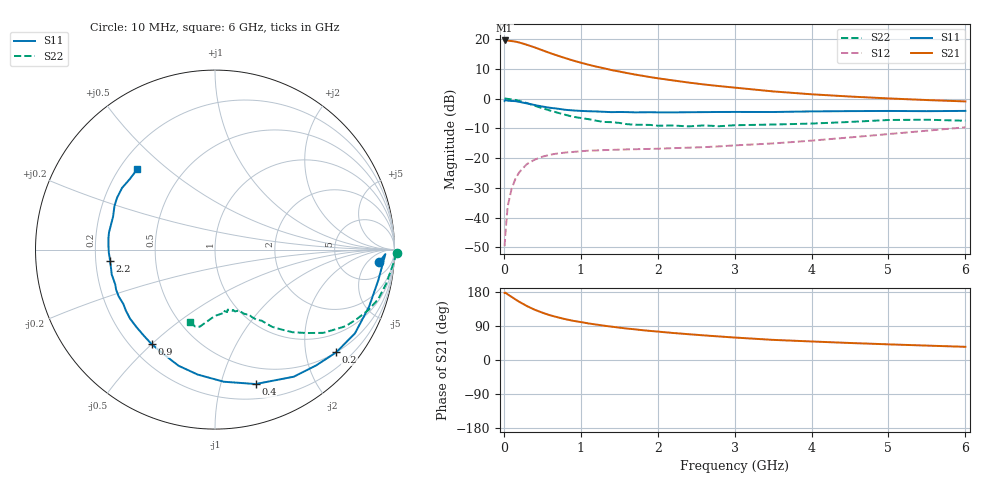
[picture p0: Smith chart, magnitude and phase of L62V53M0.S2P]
!  INFINEON TECHNOLOGIES Small Signal Semiconductors
! BFR380L3 , Si-NPN RF-Transistor in TSLP-3-1
!  Vce=2.5 V,  Ic=3 mA
! Common Emitter S-Parameters:  07. March 2005
#  GHz  S  MA  R  50
! f  S11  S21  S12  S22
! GHz  Mag  Ang  Mag  Ang  Mag  Ang  Mag  Ang
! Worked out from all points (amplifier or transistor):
!   36 points, 10 MHz to 6 GHz, reference 50 ohm
!   highest |S21| = 19.6 dB at 10 MHz (marker M1)
!   |S21| within 3 dB of that: start of sweep to 470 MHz
!   unconditionally stable (mu >= 1): 2.64 GHz to 4.677 GHz
!   at 250 MHz: K = 0.12, MSG = 20.9 dB, |S12| = -23.3 dB
!   at 1.4 GHz: K = 0.64, MSG = 13.4 dB, |S12| = -17.2 dB
!   at 6 GHz: K = 0.91, MSG = 4.4 dB, |S12| = -9.6 dB
!   S11 on the Smith chart (normalised r, x): 10 MHz: 13, -11; 200 MHz: 0.50, -2.64; 400 MHz: 0.33, -1.29; 900 MHz: 0.28, -0.50; 2.2 GHz: 0.26, -0.05; 6 GHz: 0.27, +0.40
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0.01  0.9167 -4.4  9.538 177.0  0.0033 81.0  1.014 -1.2
0.02  0.9495 -1.5  9.505 177.7  0.0053 88.8  1.005 -2.5
0.05  0.9257 -10.6  9.49 173.2  0.0154 86.5  0.9913 -5.7
0.1  0.9154 -20.3  9.312 166.7  0.0302 79.5  0.9724 -11.3
0.15  0.9087 -30.9  9.127 160.0  0.0446 73.3  0.9503 -16.9
0.2  0.8853 -40.3  8.806 153.6  0.0577 69.2  0.9189 -21.5
0.3  0.8332 -58.2  8.049 142.3  0.0794 60.1  0.8436 -30.4
0.4  0.7824 -73.2  7.292 132.8  0.0941 53.0  0.7619 -37.5
0.5  0.7378 -86.2  6.534 125.0  0.1055 48.1  0.6906 -42.3
0.6  0.7029 -97.9  5.858 118.1  0.1141 43.8  0.6315 -46.8
0.7  0.6783 -107.4  5.287 112.7  0.1197 40.9  0.5799 -50.2
0.8  0.6497 -115.9  4.808 107.7  0.1241 38.6  0.5354 -53.5
0.9  0.6339 -123.9  4.386 103.5  0.127 37.2  0.4956 -55.5
1.1  0.6147 -135.4  3.731 96.5  0.1334 35.2  0.4523 -59.5
1.3  0.6014 -145.8  3.25 90.6  0.1365 34.6  0.4061 -62.4
1.6  0.5946 -157.9  2.7 83.0  0.1402 34.8  0.3724 -67.7
2.2  0.5877 -173.9  2.027 71.3  0.147 38.9  0.3538 -74.2
2.8  0.5973 173.5  1.628 62.1  0.1576 45.3  0.3441 -82.1
3.5  0.5967 162.2  1.325 53.1  0.1766 51.4  0.3671 -88.9
4.5  0.6176 152.0  1.086 44.9  0.2229 60.0  0.4061 -96.8
5.5  0.6163 140.6  0.948 38.0  0.2892 63.0  0.4425 -104.7
6  0.6229 134.0  0.899 34.8  0.3299 62.6  0.4251 -108.8
